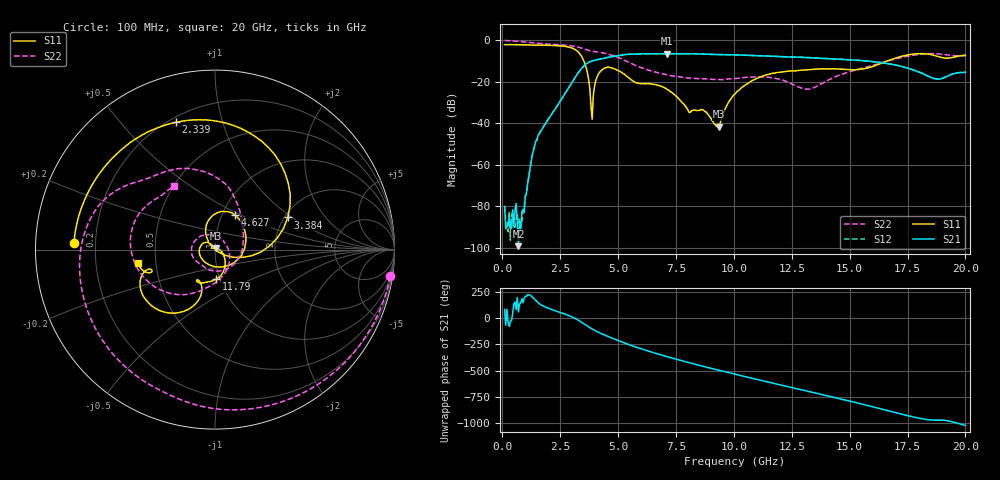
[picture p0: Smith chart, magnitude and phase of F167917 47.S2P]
!  2-Port S-parameters saved by WinCal
! VAR MeasName=S-Parameters (CALIBRATED_DATA) read from VNA (N5242A)
! VAR MeasDate=2016-11-22 9:02:07
! VAR NAME=F167917 47
! VAR FILENAME=F167917 47.S2P
! VAR DATE=2016-11-22 9:02:07
! VAR PHYS_PORTS=1,2
# Hz S DB R 50
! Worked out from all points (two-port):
!   401 points, 100 MHz to 20 GHz, reference 50 ohm
!   highest |S21| = -6.45 dB at 7.115 GHz (marker M1); lowest = -99.3 dB at 697 MHz (marker M2)
!   |S21| within 3 dB of the highest: 4.062 GHz to 14.95 GHz (10.89 GHz wide, 115 % of centre)
!   lowest |S11| = -41.7 dB at 9.354 GHz (marker M3), VSWR 1.02, Z = 50.5 + j0.651 ohm
!   |S11| at or under -10 dB: 3.522 GHz to 16.62 GHz (13.1 GHz wide, 130 % of centre)
!   |S22| runs from -23.6 to -0.1 dB; largest |S21 - S12| = 0.0046
!   S11 on the Smith chart (normalised r, x): 100 MHz: 0.12, +0.02; 2.339 GHz: 0.23, +0.72; 3.384 GHz: 2.08, +0.93; 4.627 GHz: 1.15, +0.47; 11.79 GHz: 0.96, -0.32; 20 GHz: 0.39, -0.07
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1e8  -2.09 177.3  -80.24 81.4  -79.74 124.6  -0.10 -8.7
6.97e8  -2.17 161.4  -99.30 58.6  -88.14 135.4  -0.53 -55.9
9.4575e8  -2.21 154.7  -82.96 -169.8  -79.89 -145.6  -0.78 -74.0
1.493e9  -2.31 138.7  -48.19 160.3  -48.07 160.3  -1.46 -109.0
2.33875e9  -2.60 107.0  -32.19 65.4  -32.19 65.0  -2.07 -154.2
3.3835e9  -7.06 23.8  -14.10 -34.2  -14.09 -34.1  -3.63 152.1
3.43325e9  -7.95 17.4  -13.43 -41.2  -13.43 -41.1  -3.81 149.8
3.881e9  -38.12 132.9  -9.99 -104.1  -9.94 -104.2  -5.27 133.3
4.1795e9  -15.84 104.5  -9.20 -138.3  -9.18 -138.4  -5.78 122.2
4.62725e9  -13.05 59.9  -8.11 179.0  -8.12 178.8  -6.89 101.9
5.672e9  -19.83 -72.6  -6.68 91.3  -6.67 91.3  -11.72 58.1
6.7665e9  -21.81 162.7  -6.46 15.0  -6.47 14.9  -15.84 13.8
7.11475e9  -23.67 142.4  -6.45 -7.1  -6.47 -7.2  -16.64 -6.3
8.259e9  -33.65 158.1  -6.51 -75.7  -6.53 -75.6  -18.32 -81.4
9.3535e9  -41.74 51.9  -6.90 -136.7  -6.91 -136.7  -18.96 -127.1
1.005e10  -25.90 -29.5  -7.05 -174.3  -7.07 -174.1  -18.49 -144.0
1.179125e10  -15.69 -87.4  -7.80 94.9  -7.75 95.0  -18.36 154.5
1.338325e10  -14.04 -110.6  -8.47 13.3  -8.41 13.4  -23.21 15.9
1.51245e10  -14.25 -118.8  -9.52 -76.7  -9.49 -76.8  -14.78 -88.7
1.67165e10  -9.60 -110.7  -11.35 -165.0  -11.33 -165.0  -9.81 -129.1
1.83085e10  -6.55 -151.7  -16.92 114.7  -16.73 114.1  -6.51 176.0
2e10  -7.20 -170.0  -15.50 57.9  -15.42 57.1  -7.50 122.7
